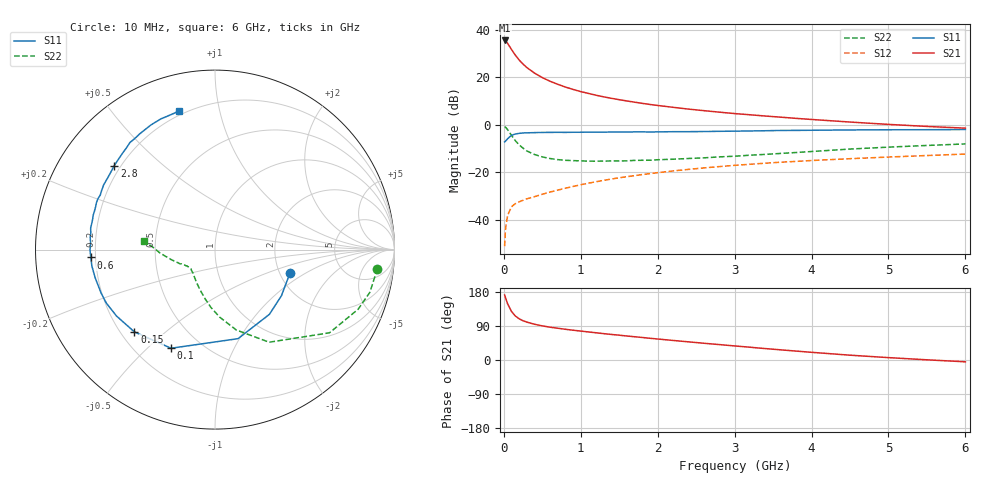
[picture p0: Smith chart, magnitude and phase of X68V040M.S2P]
! SIEMENS Small Signal Semiconductors
! BFP193W
! Si NPN RF Bipolar Junction Transistor in SOT343
! VCE = 8 V  IC = 40 mA
! Common Emitter S-Parameters:  April 1994
# GHz  S  MA  R  50
!  f  S11  S21  S12  S22
! GHz  MAG  ANG  MAG  ANG  MAG  ANG  MAG  ANG
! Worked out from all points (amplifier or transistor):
!   40 points, 10 MHz to 6 GHz, reference 50 ohm
!   highest |S21| = 35.5 dB at 10 MHz (marker M1)
!   |S21| within 3 dB of that: start of sweep to 84.1 MHz
!   unconditionally stable (mu >= 1): 766.8 MHz to 4.469 GHz
!   at 200 MHz: K = 0.48, MSG = 29.8 dB, |S12| = -32.4 dB
!   at 1.5 GHz: K = 1.11, MAG = 14.4 dB, |S12| = -22.3 dB
!   at 6 GHz: K = 0.95, MSG = 5.5 dB, |S12| = -12.3 dB
!   S11 on the Smith chart (normalised r, x): 10 MHz: 2.27, -0.73; 100 MHz: 0.34, -0.59; 150 MHz: 0.25, -0.40; 600 MHz: 0.18, -0.03; 2.8 GHz: 0.18, +0.35; 6 GHz: 0.18, +0.76
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0.01  0.4376 -17.4  59.64 171.6  0.0028 80.8  0.9112 -6.7
0.02  0.4508 -34.8  58.68 165.7  0.0058 76.1  0.895 -15.4
0.03  0.4712 -50.0  56.75 159.4  0.0081 73.6  0.864 -22.6
0.05  0.5125 -75.5  51.5 147.8  0.0126 63.2  0.7886 -36.0
0.1  0.6016 -114.0  38.48 127.9  0.0189 50.0  0.5977 -59.7
0.15  0.6418 -134.4  29.19 116.0  0.022 44.2  0.463 -75.2
0.2  0.6618 -146.0  23.03 108.7  0.0241 43.0  0.3773 -86.0
0.25  0.6748 -153.7  18.99 103.6  0.0259 43.0  0.3232 -94.0
0.3  0.6792 -159.1  16 99.9  0.0278 44.3  0.2819 -100.9
0.4  0.686 -166.9  12.22 94.3  0.0309 46.7  0.2371 -111.0
0.5  0.6921 -172.4  9.875 90.0  0.0346 49.9  0.2116 -118.7
0.6  0.6932 -176.4  8.26 86.6  0.0385 52.1  0.1958 -124.8
0.8  0.6937 177.2  6.243 81.1  0.0464 55.3  0.1795 -132.9
1.1  0.7031 170.2  4.581 74.0  0.0592 58.0  0.1722 -140.6
1.3  0.7026 165.9  3.878 69.5  0.068 58.8  0.1728 -143.4
1.6  0.7068 160.1  3.18 63.3  0.0811 58.7  0.1749 -146.7
2.2  0.7177 149.8  2.337 51.6  0.1072 56.2  0.1892 -152.9
2.8  0.7309 140.2  1.85 40.7  0.1323 52.6  0.2117 -158.1
3.2  0.7432 134.2  1.629 33.7  0.1482 49.8  0.2297 -162.5
4.5  0.7809 117.2  1.145 12.7  0.1939 40.4  0.3094 -176.8
5.5  0.7901 108.7  0.926 0.5  0.2261 34.1  0.3683 175.6
6  0.7976 104.5  0.852 -4.8  0.2428 31.3  0.3969 172.8
